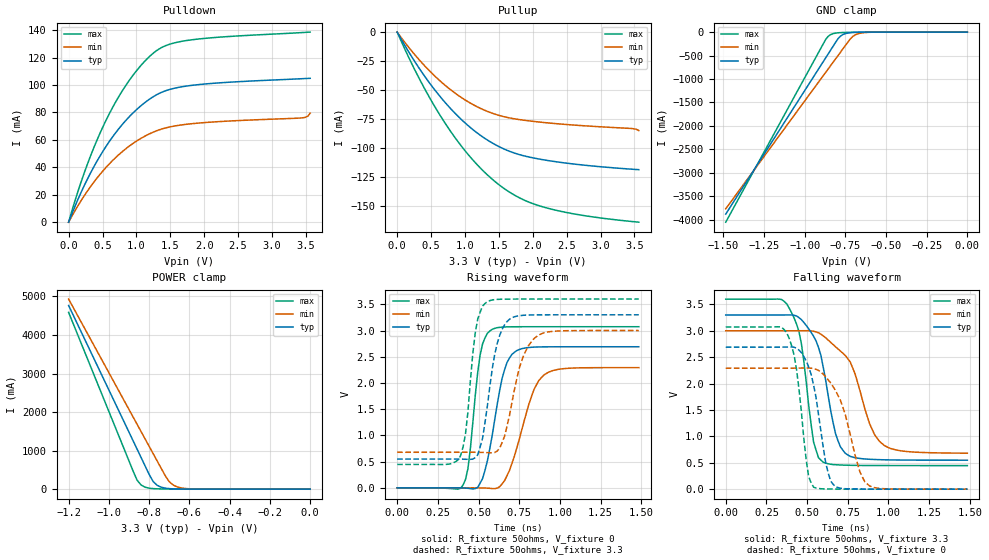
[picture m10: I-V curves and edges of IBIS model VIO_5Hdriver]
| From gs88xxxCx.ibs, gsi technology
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|  signals   DQA1-DQA9, DQB1-DQB9, DQC1-DQC9, DQD1-DQD9
[Model]   VIO_5Hdriver
Model_type   I/O
Polarity   Non-Inverting
Vinl  =   0.75v
Vinh  =   1.75v
Vmeas =   0.90v
Cref  =   0pF
Rref  =   50
Vref  =   0.90v
|  variable   typ   min   max
C_comp   3.0pF   2.5pF   3.5pF
|  variable   typ   min   max
[Temperature Range]   50   0   100
|  variable   typ   min   max
[Voltage Range]   3.3   3.0   3.6
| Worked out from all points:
|   slope of the pulldown table from 0 to 0.495 V, typ, clamps not added: 9.74 ohm
|   slope of the pullup table from 0 to 0.495 V, typ, clamps not added: 10.9 ohm
|   GND clamp passes 1 mA (typ) near -0.61 V on its own axis
|   POWER clamp passes 1 mA (typ) near -0.59 V on its own axis
|   rising waveform, R_fixture 50ohms, V_fixture 0: 20-80 % time 94.9ps typ, 132ps min, 61.9ps max; typ from 0 V to 2.69 V
|   rising waveform, R_fixture 50ohms, V_fixture 3.3: 20-80 % time 82.2ps typ, 106ps min, 59.1ps max; typ from 0.549 V to 3.3 V
|   falling waveform, R_fixture 50ohms, V_fixture 3.3: 20-80 % time 109ps typ, 164ps min, 80.3ps max; typ from 3.3 V to 0.549 V
|   falling waveform, R_fixture 50ohms, V_fixture 0: 20-80 % time 85.8ps typ, 132ps min, 67.7ps max; typ from 2.69 V to 0 V
[Pulldown]
| voltage   typ   min   max
0V        -445.6pA   -1.181nA   -285.9pA
144mV     17.32mA    12.5mA     23.36mA
288mV     32.45mA    23.45mA    43.7mA
576mV     57.05mA    41.24mA    76.69mA
900mV     77.16mA    55.66mA    103.8mA
1.08V     85.43mA    61.48mA    115mA
1.26V     91.83mA    65.9mA     123.7mA
1.476V    96.57mA    69.27mA    129.5mA
1.8V      99.66mA    71.72mA    132.9mA
3.42V     104.6mA    75.95mA    138.2mA
3.528V    104.8mA    77.28mA    138.5mA
3.564V    104.9mA    79.49mA    138.6mA
[Pullup]
| voltage (VDDQ-Vout)   typ   min   max
0V        394.9pA    1.311nA    168.6pA
180mV     -18mA      -13.84mA   -22.97mA
360mV     -34.21mA   -26.17mA   -43.86mA
720mV     -61.49mA   -46.47mA   -79.62mA
1.08V     -82.23mA   -61.2mA    -107.7mA
1.26V     -90.25mA   -66.56mA   -119.1mA
1.476V    -97.89mA   -71.3mA    -130.3mA
1.8V      -105.5mA   -75.35mA   -142.7mA
2.196V    -110.4mA   -78.08mA   -151.4mA
2.772V    -114.7mA   -80.77mA   -158.2mA
3.456V    -118.1mA   -83.07mA   -163.2mA
3.564V    -118.5mA   -84.81mA   -163.8mA
[GND Clamp]
| voltage   typ   min   max
-1.485V   -3.884A    -3.771A    -4.056A
-885mV    -626.9mA   -926.9mA   -247.2mA
-870mV    -545.6mA   -856mA     -153.5mA
-855mV    -464.4mA   -785mA     -89.11mA
-825mV    -301.9mA   -643.2mA   -32.88mA
-795mV    -141.5mA   -501.4mA   -15.38mA
-780mV    -86.61mA   -430.5mA   -11.65mA
-750mV    -32.85mA   -288.8mA   -7.734mA
-705mV    -8.727mA   -95.28mA   -4.834mA
-660mV    -2.907mA   -24.97mA   -2.925mA
-555mV    -316.7uA   -1.176mA   -484.9uA
0V        -445.6pA   -1.181nA   -285.9pA
[POWER Clamp]
| voltage (VDDQ-Vout)   typ   min   max
-1.2V     4.765A     4.931A     4.585A
-880mV    1.258A     1.875A     474.1mA
-860mV    1.039A     1.684A     234.3mA
-840mV    820.4mA    1.493A     107.4mA
-820mV    601.5mA    1.302A     50.64mA
-780mV    197.3mA    920.5mA    14.28mA
-760mV    99.71mA    729.7mA    9.034mA
-720mV    26.23mA    348.2mA    4.898mA
-700mV    13.96mA    192.6mA    3.916mA
-660mV    4.495mA    57.55mA    2.579mA
-560mV    510.5uA    2.941mA    648.3uA
0V        395pA      1.311nA    168.9pA
[Ramp]
| voltage   typ   min   max
dV/dt_r   0.74/187p   0.51/270p   0.95/124p
dV/dt_f   0.87/155p   0.71/182p   1.02/128p
R_load  =   50ohms
[Rising Waveform]
C_fixture =   0.0pF
R_fixture =   50ohms
V_fixture =   0
| Time   V(typ)   V(min)   V(max)
0s        3.002nV    10.49nV    1.477nV
405ps     -1.339mV   337.9uV    53.33mV
435ps     -8.304mV   467.3uV    369.7mV
510ps     91.48mV    -559.7uV   2.535V
585ps     1.017V     -13.21mV   3.025V
645ps     2.089V     76.81mV    3.066V
690ps     2.474V     331.3mV    3.071V
840ps     2.683V     1.868V     3.073V
900ps     2.689V     2.147V     3.073V
1.485ns   2.691V     2.293V     3.073V
[Rising Waveform]
C_fixture =   0.0pF
R_fixture =   50ohms
V_fixture =   3.3
V_fixture_min =  3.0
V_fixture_max =  3.6
| Time   V(typ)   V(min)   V(max)
0s        548.9mV    679.1mV    446.9mV
390ps     547.7mV    679.4mV    615.4mV
420ps     545.2mV    679.5mV    1.032V
480ps     577.3mV    678.9mV    2.957V
555ps     1.575V     671.6mV    3.555V
600ps     2.551V     675.2mV    3.59V
645ps     3.023V     865.9mV    3.598V
750ps     3.282V     2.28V      3.6V
840ps     3.298V     2.844V     3.6V
1.485ns   3.3V       3V         3.6V
[Falling Waveform]
C_fixture =   0.0pF
R_fixture =   50ohms
V_fixture =   3.3
V_fixture_min =  3.0
V_fixture_max =  3.6
| Time   V(typ)   V(min)   V(max)
0s        3.3V       3V         3.6V
375ps     3.301V     3V         3.51V
450ps     3.25V      3.001V     2.988V
540ps     2.897V     2.992V     892.5mV
600ps     2.299V     2.902V     508.2mV
675ps     1.052V     2.697V     463.3mV
750ps     648.8mV    2.474V     453.5mV
885ps     566.3mV    1.234V     448.3mV
975ps     556.5mV    827.2mV    447.4mV
1.485ns   549.1mV    681.7mV    446.9mV
[Falling Waveform]
C_fixture =   0.0pF
R_fixture =   50ohms
V_fixture =   0
| Time   V(typ)   V(min)   V(max)
0s        2.691V     2.293V     3.073V
375ps     2.693V     2.292V     2.963V
420ps     2.689V     2.293V     2.542V
495ps     2.428V     2.296V     545.4mV
540ps     1.972V     2.284V     38.17mV
615ps     490.4mV    2.129V     4.365mV
675ps     45.34mV    1.868V     1.824mV
825ps     2.187mV    325.1mV    328.2uV
885ps     1.213mV    59.72mV    164.2uV
1.485ns   6.438uV    102.7uV    768.2nV
